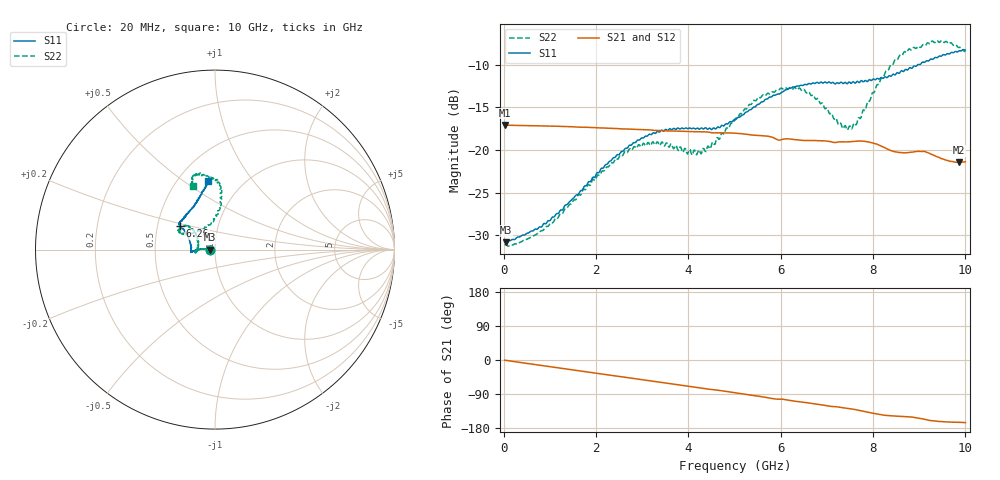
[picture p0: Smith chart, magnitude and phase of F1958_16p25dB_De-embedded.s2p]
! Integrated Device Technology
! Corporate Headquarters
! 6024 Silver Creek Valley Road
! San Jose, CA 95138  USA
! Phone:  1-408-284-8200
! Toll Free:  1-800-223-1366
! Webpage:  http://www.idt.com/
! Timing and RF Division
! 515 Groton Road, Suite 102
! Westford, MA 01886-6024
! Device:  F1958
! Description: 7-bit 0.25 dB Digital Step Attenuator
! Frequency:  0.001 -  6.000 GHz
! Package:  4x4 mm Thin QFN Plastic Package: 24 pin
! Ports:  2 RF, 12 DC
!  Pin  1  = D0
!  Pin  2  = VDD
!  Pin  3  = VMODE
!  Pin  4  = GND
!  Pin  5  = RF1  =  Port 1
!  Pin  6  = GND
!  Pin  7  = GND
!  Pin  8  = GND
!  Pin  9  = GND
!  Pin 10  = GND
!  Pin 11  = GND
!  Pin 12  = GND
!  Pin 13  = GND
!  Pin 14  = RF2  =  Port 2
!  Pin 15  = GND
!  Pin 16  = LE
!  Pin 17  = CLK
!  Pin 18  = DATA
!  Pin 19  = D6
!  Pin 20  = D5
!  Pin 21  = D4
!  Pin 22  = D3
!  Pin 23  = D2
!  Pin 24  = D1
! State:  65
! Atten State:  16.25 dB
! Voltage:  +3.30 Volts
! Current:  0.258 mA
! Data:  The device was measured on a F1958 evaluation board which has
!  individual transmission lines to the RF pins.  Data was collected
!  using a calibrated network analyzer.  The evaluation board was
!  de-embedded using Automatic Fixture Removal (AFR).
!  The reference plane is the edge of the package pin.
! Misc:
!  Action Tracker AT0419
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# GHz S dB R 50
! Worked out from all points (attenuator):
!   500 points, 20 MHz to 10 GHz, reference 50 ohm
!   highest |S21| = -17.08 dB at 20 MHz (marker M1); lowest = -21.5 dB at 9.86 GHz (marker M2)
!   lowest |S11| = -30.8 dB at 40 MHz (marker M3), VSWR 1.06, Z = 47.2 - j0.0701 ohm
!   |S11| at or under -10 dB: start of sweep to 8.974 GHz; 9.013738 GHz to 9.020733 GHz (6.995 MHz wide, 0.0776 % of centre)
!   |S22| runs from -31.3 to -7.2 dB; largest |S21 - S12| = 0.00044
!   S11 on the Smith chart (normalised r, x): 20 MHz: 0.94, -0.00; 6.26 GHz: 0.66, +0.18; 10 GHz: 0.69, +0.62
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0.02  -30.77 -178.5  -17.08 -0.5  -17.08 -0.4  -31.11 -178.7
0.04  -30.79 -178.5  -17.09 -0.8  -17.09 -0.8  -31.07 -178.1
0.32  -30.19 177.3  -17.13 -5.8  -17.13 -5.8  -30.96 177.0
0.84  -28.87 175.3  -17.19 -14.9  -17.18 -14.9  -29.43 176.5
1.7  -24.71 176.4  -17.34 -29.8  -17.33 -29.8  -24.88 175.6
2.62  -19.89 -179.3  -17.54 -45.7  -17.52 -45.7  -20.22 -178.1
2.92  -18.84 -176.6  -17.60 -50.8  -17.59 -50.9  -19.38 -175.4
3.36  -17.89 -174.1  -17.73 -58.4  -17.72 -58.5  -19.33 -171.0
4.24  -17.57 -179.2  -17.87 -73.1  -17.88 -73.2  -20.05 167.3
4.5  -17.62 174.8  -17.98 -77.9  -17.99 -78.0  -19.43 152.0
5.02  -16.47 160.5  -18.04 -86.6  -18.05 -86.6  -16.29 138.8
5.54  -14.62 150.3  -18.31 -95.9  -18.32 -95.9  -13.85 140.1
6.26  -12.63 146.1  -18.76 -107.8  -18.77 -107.8  -12.88 150.8
6.68  -12.20 144.0  -18.90 -114.6  -18.91 -114.5  -13.61 153.2
7.3  -12.06 137.5  -19.05 -125.0  -19.05 -124.9  -16.85 132.4
7.5  -12.10 134.6  -19.04 -128.6  -19.05 -128.5  -17.20 114.5
7.7  -12.13 130.5  -18.95 -132.9  -18.96 -132.8  -16.21 98.3
8.34  -11.33 115.5  -19.96 -147.0  -19.96 -147.1  -10.57 82.8
8.68  -10.70 108.8  -20.33 -149.0  -20.33 -149.0  -8.48 87.1
9.26  -9.35 100.9  -20.51 -159.9  -20.51 -159.9  -7.37 99.6
9.86  -8.41 96.2  -21.45 -164.4  -21.48 -164.3  -8.01 108.2
10  -8.30 96.2  -21.37 -165.4  -21.40 -165.2  -8.51 108.9
